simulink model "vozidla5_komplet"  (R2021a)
settings: Solver=VariableStepAuto  StartTime=0.0  StopTime=120  RelTol=1e-9
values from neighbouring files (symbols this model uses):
  A = A(1:(pocet_stavu),1:(pocet_stavu))    [appDekompLQR.m]    (also in appLQR.m = A(1:(2*N-1),1:(2*N-1)); appSYM.m = A(1:(2*N-1),1:(2*N-1)); appSZV.m = A(1:(2*N-1),1:(2*N-1)); central_LQR.m = A(1:(2*N-1),1:(2*N-1)))
  B = zeros(pocet_stavu,N)    [appDekompLQR.m]    (also in appLQR.m = zeros(2*N-1,N); appSYM.m = zeros(2*N-1,N); appSZV.m = zeros(2*N-1,N); central_LQR.m = zeros(2*N-1,N))
  C = eye(pocet_stavu)    [appDekompLQR.m]    (also in appLQR.m; appSYM.m; appSZV.m; central_LQR.m)
  conds0 = zeros(1,2*N-1)    [central_LQR.m]    (also in central_SYM.m; distri_STRUKTURAL.m = zeros(1,pocet_stavu); distri_SZV.m; porovnani_rizeni.m)
  D = zeros(pocet_stavu,N)    [appDekompLQR.m]    (also in appLQR.m; appSYM.m; appSZV.m; central_LQR.m)
  K = zeros(N,pocet_stavu)    [appDekompLQR.m]    (also in appSYM.m = [[0,-1/5,0,-3/20,0,-1/10,0,-1/20,0]; appSZV.m = [[-5/2,-3,7/4,1/2,0,0,0];[-1/7,-2/7,-7/2,-37/7,18/7,0,0];[0,; central_LQR.m = -K; central_SYM.m = [[0,-1/5,0,-3/20,0,-1/10,0,-1/20,0])

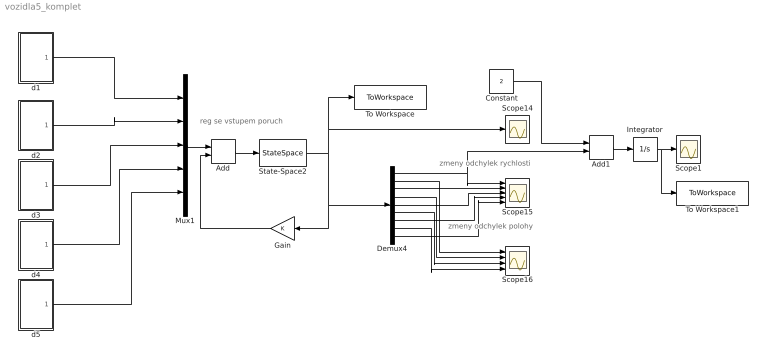
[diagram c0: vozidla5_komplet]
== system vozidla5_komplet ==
  note: zmeny odchylek polohy
  note: zmeny odchylek rychlosti
  note: reg se vstupem poruch
  Add : Sum
  Add1 : Sum
  Constant : Constant  Value=2
  Demux4 : Demux  Outputs=9
  Gain : Gain  Gain=K  Multiplication=Matrix(K*u)
  Integrator : Integrator
  Mux1 : Mux  Inputs=5
  Scope1 : Scope
  Scope14 : Scope
  Scope15 : Scope  NumInputPorts=5
  Scope16 : Scope  NumInputPorts=4
  State-Space2 : StateSpace  A=A  B=B  C=C  D=D  InitialCondition=conds0
  To Workspace : ToWorkspace  VariableName=vystup  SaveFormat=Structure  SampleTime=-1
  To Workspace1 : ToWorkspace  VariableName=vystup1  SaveFormat=Structure  SampleTime=-1
  d1 : Subsystem
  d2 : Subsystem
  d3 : Subsystem
  d4 : Subsystem
  d5 : Subsystem
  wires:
  Demux4/6 -> Scope16/3
  Demux4/4 -> Scope16/2
  Demux4/7 -> Scope15/4
  Demux4/8 -> Scope16/4
  Demux4/2 -> Scope16/1
  Demux4/3 -> Scope15/2
  Demux4/9 -> Scope15/5
  Demux4/5 -> Scope15/3
  Demux4/1 -> Add1/2, Scope15/1
  Mux1/1 -> Add/1
  Gain/1 -> Add/2
  State-Space2/1 -> Demux4/1, Gain/1, Scope14/1, To Workspace/1
  Add/1 -> State-Space2/1
  d1/1(Out1) -> Mux1/1
  d2/1(Out1) -> Mux1/2
  d3/1(Out1) -> Mux1/3
  d4/1(Out1) -> Mux1/4
  d5/1(Out1) -> Mux1/5
  Constant/1 -> Add1/1
  Add1/1 -> Integrator/1
  Integrator/1 -> To Workspace1/1, Scope1/1

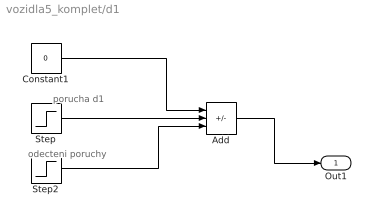
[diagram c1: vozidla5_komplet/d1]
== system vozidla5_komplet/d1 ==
  note: odecteni poruchy
  note: porucha d1
  Add : Sum  Inputs=++-
  Constant1 : Constant  Value=0
  Step : Step  Time=5  After=2  SampleTime=0
  Step2 : Step  Time=6  After=2  SampleTime=0
  Out1 : Outport
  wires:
  Constant1/1 -> Add/1
  Step2/1 -> Add/3
  Add/1 -> Out1/1
  Step/1 -> Add/2

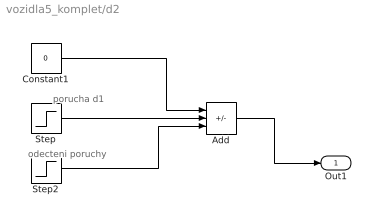
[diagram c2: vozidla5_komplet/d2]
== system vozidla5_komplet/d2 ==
  note: odecteni poruchy
  note: porucha d1
  Add : Sum  Inputs=++-
  Constant1 : Constant  Value=0
  Step : Step  Time=25  After=2  SampleTime=0
  Step2 : Step  Time=26  After=2  SampleTime=0
  Out1 : Outport
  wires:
  Constant1/1 -> Add/1
  Step2/1 -> Add/3
  Add/1 -> Out1/1
  Step/1 -> Add/2

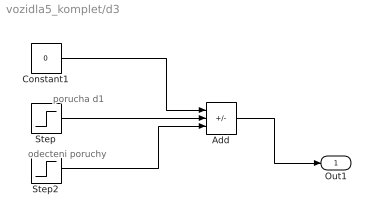
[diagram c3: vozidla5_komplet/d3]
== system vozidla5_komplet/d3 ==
  note: odecteni poruchy
  note: porucha d1
  Add : Sum  Inputs=++-
  Constant1 : Constant  Value=0
  Step : Step  Time=45  After=2  SampleTime=0
  Step2 : Step  Time=46  After=2  SampleTime=0
  Out1 : Outport
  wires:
  Constant1/1 -> Add/1
  Step2/1 -> Add/3
  Add/1 -> Out1/1
  Step/1 -> Add/2

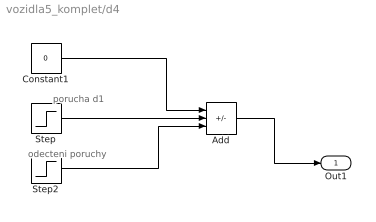
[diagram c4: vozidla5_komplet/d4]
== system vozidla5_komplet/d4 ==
  note: odecteni poruchy
  note: porucha d1
  Add : Sum  Inputs=++-
  Constant1 : Constant  Value=0
  Step : Step  Time=65  After=2  SampleTime=0
  Step2 : Step  Time=66  After=2  SampleTime=0
  Out1 : Outport
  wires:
  Constant1/1 -> Add/1
  Step2/1 -> Add/3
  Add/1 -> Out1/1
  Step/1 -> Add/2

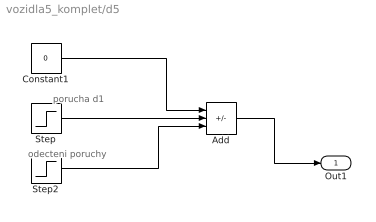
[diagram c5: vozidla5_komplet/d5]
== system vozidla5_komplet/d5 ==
  note: odecteni poruchy
  note: porucha d1
  Add : Sum  Inputs=++-
  Constant1 : Constant  Value=0
  Step : Step  Time=85  After=2  SampleTime=0
  Step2 : Step  Time=86  After=2  SampleTime=0
  Out1 : Outport
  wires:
  Constant1/1 -> Add/1
  Step2/1 -> Add/3
  Add/1 -> Out1/1
  Step/1 -> Add/2
